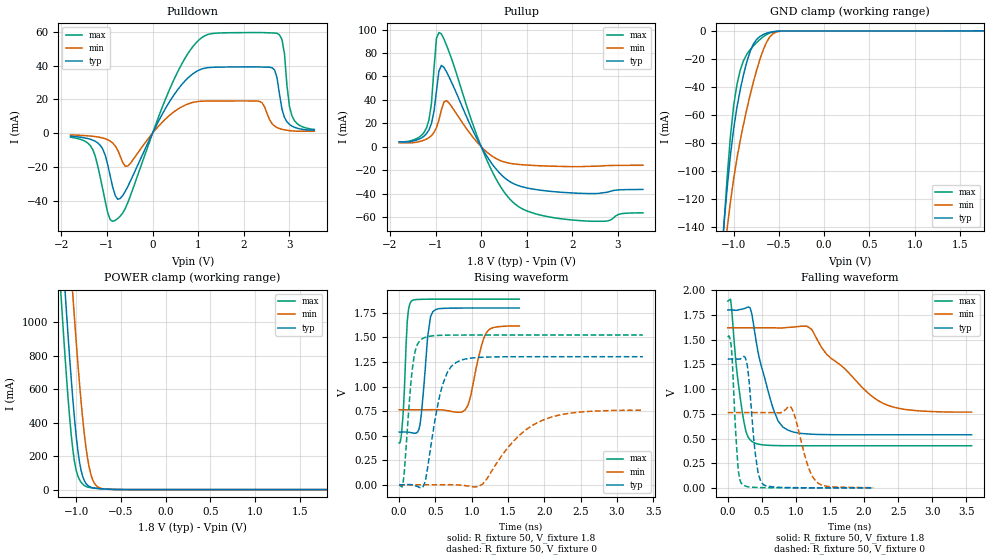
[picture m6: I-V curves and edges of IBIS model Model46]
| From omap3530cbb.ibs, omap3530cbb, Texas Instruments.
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| Model based on original model for BQOMAPPROGIOCSHYFBPB_7LM
|   Sub model MODE01_PU_ON_1P8
[model]   Model46
|[Input Load]   PU
|[Output Drive] DS01
|Voltage   1.8V
|Mode   I/O
Model_type   I/O
Polarity   Non-Inverting
Enable   Active-Low
Vinl =  0.63
Vinh =  1.17
Cref =  15.0000pF
Rref =  100.0000M
Vref =  0V
Vmeas =  0.9
C_comp   0.8864943p   0.7714798p   1.034566p
[Model Spec]
Vinl   0.63   0.567   0.6615
Vinh   1.17   1.053   1.2285
[Temperature Range]   25   125   -40
[Voltage Range]   1.8   1.62   1.89
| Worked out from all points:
|   slope of the pulldown table from 0 to 0.27 V, typ, clamps not added: 19.3 ohm
|   slope of the pullup table from 0 to 0.27 V, typ, clamps not added: 16.6 ohm
|   GND clamp passes 1 mA (typ) near -0.60 V on its own axis
|   POWER clamp passes 1 mA (typ) near -0.55 V on its own axis
|   rising waveform, R_fixture 50, V_fixture 1.8: 20-80 % time 86.5ps typ, 154ps min, 53.3ps max; typ from 0.538 V to 1.8 V
|   rising waveform, R_fixture 50, V_fixture 0: 20-80 % time 201ps typ, 558ps min, 101ps max; typ from 0.001 V to 1.3 V
|   falling waveform, R_fixture 50, V_fixture 1.8: 20-80 % time 272ps typ, 743ps min, 144ps max; typ from 1.8 V to 0.538 V
|   falling waveform, R_fixture 50, V_fixture 0: 20-80 % time 105ps typ, 187ps min, 69.7ps max; typ from 1.3 V to 0.001 V
[POWER_clamp]
-1.8V     7.429A     8.065A     7.064A
-1.182V   1.663A     2.35A      1.259A
-1.164V   1.508A     2.193A     1.106A
-1.127V   1.206A     1.883A     813.3mA
-1.073V   782.1mA    1.435A     426.4mA
-1.036V   530.7mA    1.15A      232.5mA
-981.8mV  234.7mA    756.4mA    81.82mA
-909.1mV  52.91mA    331.4mA    24.57mA
-872.7mV  25.71mA    185.5mA    15.52mA
-818.2mV  11.31mA    62.04mA    10.16mA
-709.1mV  4.634mA    6.205mA    4.543mA
1.8V      403.3pA    2.083nA    554.5pA
[Pulldown]
-1.8V     -1.789mA   -1.059mA   -2.429mA
-1.364V   -3.636mA   -1.733mA   -7.448mA
-1.145V   -7.295mA   -2.547mA   -26.48mA
-818.2mV  -36.98mA   -7.617mA   -51.58mA
-545.5mV  -31.67mA   -19.52mA   -41.22mA
654.5mV   29.22mA    15.79mA    41.66mA
1.527V    39.09mA    19.05mA    59.31mA
2.345V    39.14mA    18.78mA    59.5mA
2.618V    38.71mA    5.636mA    59.27mA
2.782V    23.04mA    2.689mA    58.16mA
3.055V    4.158mA    1.352mA    10.28mA
3.545V    1.801mA    1.153mA    2.203mA
[Pullup]
-1.8V     3.998mA    3.315mA    4.26mA
-1.2V     11.17mA    6.515mA    16.06mA
-1.091V   19.96mA    9.525mA    37.21mA
-1.036V   30.02mA    12.16mA    66.25mA
-981.8mV  47.48mA    16.29mA    92.64mA
-927.3mV  64.65mA    22.8mA     97.4mA
-872.7mV  69.46mA    31.49mA    96.17mA
-763.6mV  64.03mA    39.31mA    86.78mA
54.55mV   -3.696mA   -2.123mA   -5.184mA
709.1mV   -31.49mA   -14.6mA    -47.81mA
2.127V    -39.64mA   -17mA      -62.9mA
3.545V    -36.43mA   -15.79mA   -56.35mA
[GND_clamp]
-1.8V     -794.1mA   -670.5mA   -980.8mA
-1.109V   -139.6mA   -162.6mA   -140.1mA
-1.073V   -112.8mA   -141.5mA   -105.3mA
-1.036V   -89.25mA   -122.4mA   -75.78mA
-1V       -69.85mA   -105.6mA   -53.39mA
-963.6mV  -54.51mA   -91mA      -38.25mA
-890.9mV  -31.23mA   -66.63mA   -21.22mA
-818.2mV  -14.77mA   -45.89mA   -13.43mA
-709.1mV  -3.956mA   -20.2mA    -6.107mA
-600mV    -995.8uA   -4.202mA   -1.492mA
-490.9mV  -212.7uA   -380.9uA   -249.1uA
1.764V    -5.644uA   14.27uA    -26.63uA
[Ramp]
dV/dt_f  0.7756806/0.2727978n  0.5241662/0.7536241n  0.9039889/0.1451597n
dV/dt_r  0.8010481/0.2014172n   0.470664/0.5679735n  0.9365271/0.1016929n
R_load = 50
[Rising Waveform]
R_fixture = 50
V_fixture = 1.8
V_fixture_min = 1.62
V_fixture_max = 1.89
0s        537.7mV    764.1mV    426.8mV
56ps      538.4mV    764.1mV    738.7mV
112ps     537.5mV    764.1mV    1.664V
168ps     531.2mV    764mV      1.869V
288ps     614.4mV    764mV      1.888V
392ps     1.5V       764.9mV    1.889V
464ps     1.762V     765.3mV    1.89V
912ps     1.799V     764mV      1.89V
1.2ns     1.8V       1.546V     1.89V
1.656ns   1.8V       1.617V     1.89V
[Rising Waveform]
R_fixture = 50
V_fixture = 0
V_fixture_min = 0
V_fixture_max = 0
0s        1.325mV    844.3uV    1.567mV
64ps      1.971mV    846.9uV    78.12mV
160ps     2.918mV    847.3uV    1.019V
208ps     -4.394mV   844.3uV    1.315V
312ps     -29.99mV   751.9uV    1.484V
576ps     957.4mV    1.71mV     1.522V
784ps     1.245V     1.124mV    1.524V
1.152ns   1.299V     9.472mV    1.525V
2.024ns   1.304V     671.7mV    1.525V
3.36ns    1.304V     759.3mV    1.525V
[Falling Waveform]
R_fixture = 50
V_fixture = 1.8
V_fixture_min = 1.62
V_fixture_max = 1.89
0s        1.8V       1.62V      1.89V
48ps      1.8V       1.62V      1.869V
128ps     1.797V     1.62V      1.215V
240ps     1.813V     1.62V      658mV
376ps     1.664V     1.62V      461.2mV
664ps     806.8mV    1.62V      429.6mV
880ps     585.8mV    1.623V     427.3mV
1.232ns   543.7mV    1.604V     426.9mV
2.272ns   537.8mV    858.1mV    426.8mV
3.576ns   537.7mV    767.4mV    426.8mV
[Falling Waveform]
R_fixture = 50
V_fixture = 0
V_fixture_min = 0
V_fixture_max = 0
0s        1.304V     762.6mV    1.525V
56ps      1.304V     762.6mV    1.394V
152ps     1.303V     762.6mV    201.2mV
216ps     1.323V     762.6mV    33.86mV
296ps     1.19V      762.6mV    11.86mV
448ps     142.5mV    762.6mV    4.991mV
528ps     30.99mV    762.7mV    3.554mV
928ps     3.964mV    818.6mV    1.67mV
1.32ns    1.704mV    52.01mV    1.573mV
2.136ns   1.338mV    4.128mV    1.567mV
